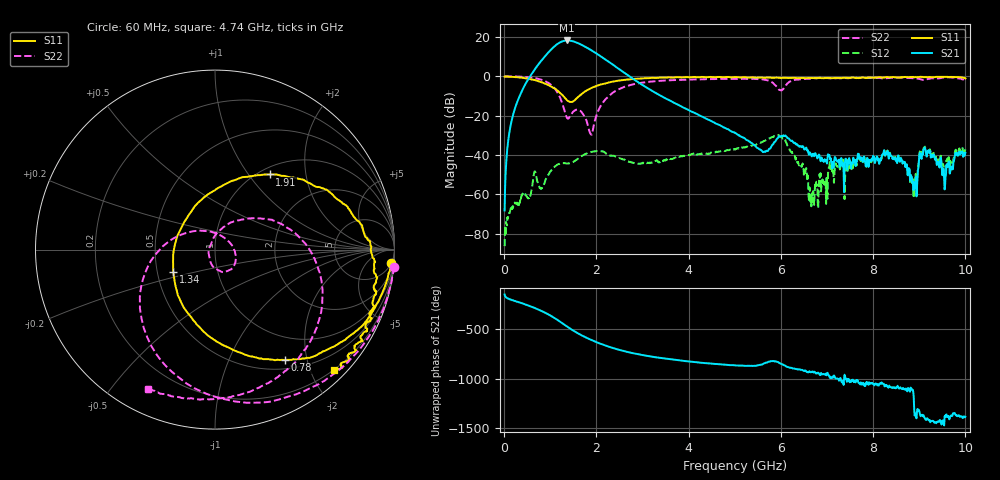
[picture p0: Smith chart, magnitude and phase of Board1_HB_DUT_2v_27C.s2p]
! Created Tue May 27 10:45:08 2025
# hz S ma R 50
! 2 Port Network Data from SP1.SP block
! freq  magS11  angS11  magS21  angS21  magS12  angS12  magS22  angS22
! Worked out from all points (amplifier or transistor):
!   1000 points, 10 MHz to 10 GHz, reference 50 ohm
!   highest |S21| = 18.3 dB at 1.36 GHz (marker M1)
!   |S21| within 3 dB of that: 1.091 GHz to 1.742 GHz (651.5 MHz wide, 46 % of centre)
!   unconditionally stable (mu >= 1): 58.56 MHz to 62.32 MHz; 89.09 MHz to 108.1 MHz; 112 MHz to end of sweep
!   at 1.67 GHz: K = 7.39, MAG = 16.8 dB, |S12| = -40.7 dB
!   at 5.01 GHz: K = 18.01, MAG = -11.5 dB, |S12| = -37.0 dB
!   at 10 GHz: K = 222.38, MAG = -27.4 dB, |S12| = -37.1 dB
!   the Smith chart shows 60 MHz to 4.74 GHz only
!   S11 on the Smith chart (normalised r, x): 60 MHz: 6, -25; 780 MHz: 0.62, -1.64; 1.34 GHz: 0.61, -0.16; 1.91 GHz: 1.11, +1.27; 4.74 GHz: 0.19, -2.39
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1e7  0.9808 -1.0  0.0003863 -156.3  4.78e-05 118.3  1.005 -0.8
6e7  0.9831 -4.3  0.01124 168.6  0.0001614 102.9  0.9994 -5.5
5.1e8  0.8744 -35.9  0.7992 95.9  0.0008085 88.2  0.9518 -50.2
7.8e8  0.7283 -57.8  2.298 45.1  0.001417 81.8  0.8389 -85.5
9.5e8  0.6082 -74.1  3.968 6.0  0.003057 116.8  0.6915 -115.1
1.11e9  0.4786 -95.0  6.072 -37.4  0.005207 99.9  0.4676 -152.2
1.24e9  0.3553 -121.1  7.59 -77.8  0.00615 82.9  0.2391 164.8
1.34e9  0.2635 -152.1  8.153 -110.1  0.00606 74.9  0.1013 101.8
1.36e9  0.2482 -160.2  8.183 -116.5  0.006061 74.8  0.0895 82.2
1.51e9  0.2352 131.8  7.683 -161.8  0.006752 76.2  0.1295 -27.8
1.68e9  0.3549 84.1  6.323 153.7  0.009363 69.2  0.1219 -77.0
1.91e9  0.5178 54.0  4.455 103.0  0.01204 45.0  0.03537 131.6
2.27e9  0.6999 28.6  2.333 39.5  0.009654 9.6  0.3155 33.0
2.66e9  0.8288 9.4  1.109 -11.8  0.007139 -2.4  0.5664 -7.0
3.34e9  0.9181 -14.4  0.3482 -70.2  0.006598 10.6  0.762 -52.1
4.74e9  0.9441 -45.2  0.05161 -140.0  0.01244 -4.1  0.8604 -115.8
5.01e9  0.9617 -50.3  0.03587 -148.3  0.0141 -10.3  0.8642 -126.3
6e9  0.9068 -70.3  0.03003 -131.7  0.02865 -103.9  0.4369 -150.1
6.67e9  0.907 -90.5  0.009186 148.2  0.001051 -62.2  0.8863 -156.2
8.34e9  0.9409 -136.7  0.008024 -3.9  0.008341 -10.2  0.9066 167.2
8.9e9  0.9521 -147.5  0.001786 67.7  0.002364 65.4  0.8963 155.0
1e10  0.887 -164.9  0.01137 55.9  0.01395 55.1  0.8185 137.9
